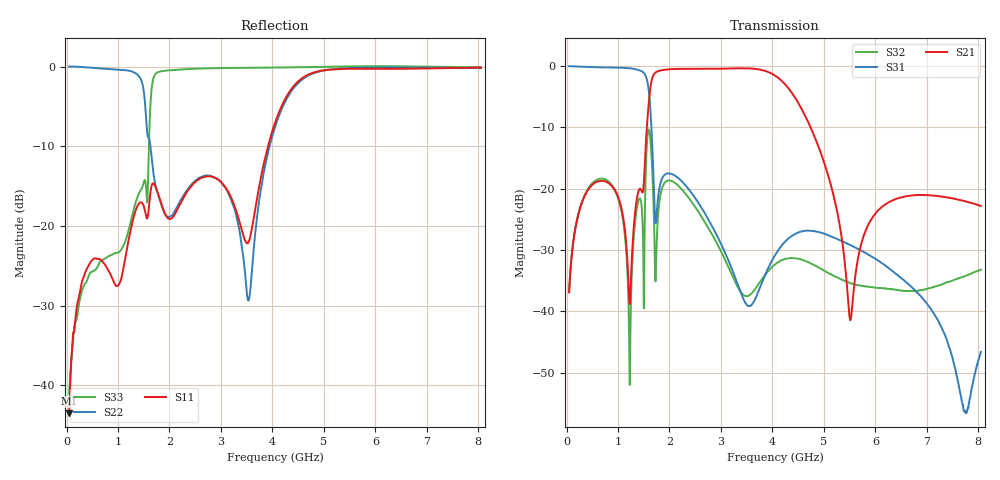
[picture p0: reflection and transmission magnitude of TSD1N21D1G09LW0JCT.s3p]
# MHZ S RI R 50
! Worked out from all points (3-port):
!   1601 points, 50 MHz to 8.05 GHz, reference 50 ohm
!   strongest paths, dB at 50 MHz, 2.05 GHz, 4.05 GHz, 6.05 GHz, 8.05 GHz:
!     S21: -36.9, -0.5, -1.5, -23.5, -22.8
!     S31: 0.0, -17.6, -30.8, -31.7, -46.6
!     S32: -36.8, -18.7, -32.3, -36.2, -33.2
!   lowest |S11| = -43.5 dB at 50 MHz (marker M1), VSWR 1.01, Z = 49.9 - j0.651 ohm
!   |S11| at or under -10 dB: start of sweep to 3.914 GHz
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50  -0.00145 -0.00653  0.00116 0.0143  0.9934 -0.063
    0.00114 0.0143  0.9905 -0.1438  0.00189 0.0142
    0.9975 -0.0629  0.0019 0.0143  0.00689 -0.00561
580  -0.0536 -0.0323  0.0848 0.0757  0.7352 -0.6481
     0.0844 0.0762  -0.0079 -0.9777  0.1172 0.00977
     0.7364 -0.6473  0.1173 0.00935  -0.00262 -0.0538
1150  0.0608 0.0236  0.0382 0.0113  -0.0718 -0.9641
      0.0381 0.0114  -0.9458 -0.0768  0.00107 -0.035
      -0.0727 -0.9647  0.000886 -0.0351  0.0607 -0.0545
1510  -0.0985 -0.0847  -0.1277 -0.0117  -0.8446 -0.2193
      -0.1282 -0.0117  0.5781 0.3214  -0.0163 0.0166
      -0.8465 -0.2173  -0.0162 0.0166  0.1893 -0.0327
1885  0.0193 -0.1239  0.1702 0.9159  -0.0925 -0.0866
      0.1699 0.9162  0.0675 0.1047  0.0995 -0.0414
      -0.0931 -0.0867  0.0998 -0.0419  0.6203 -0.7056
3530  0.0397 -0.068  0.6828 -0.6725  -0.00519 0.00972
      0.6826 -0.6737  -0.0319 0.0121  -0.0019 -0.0132
      -0.00527 0.00976  -0.00188 -0.0133  -0.4763 -0.8596
4050  0.3824 -0.2248  0.0323 -0.8375  0.0245 0.0154
      0.0334 -0.837  0.3864 0.1567  -0.00388 -0.024
      0.0243 0.0153  -0.00389 -0.0239  -0.6236 -0.7632
5515  -0.5715 -0.7816  -0.00113 -0.00845  0.0275 -0.0219
      -0.00111 -0.00844  0.1068 -0.9741  -0.0161 0.00598
      0.0271 -0.0218  -0.0159 0.00609  -0.7539 -0.661
6125  -0.8325 -0.4938  0.0597 -0.0394  0.0169 -0.0179
      0.0595 -0.0387  -0.0926 -0.9849  -0.0129 0.00818
      0.0172 -0.0179  -0.0131 0.0083  -0.7273 -0.6949
8050  -0.9512 0.2584  0.0394 -0.0605  -0.000189 0.0047
      0.0388 -0.0612  -0.2208 -0.9538  -0.0192 0.011
      -0.000106 0.00468  -0.019 0.0109  -0.7165 -0.6825
